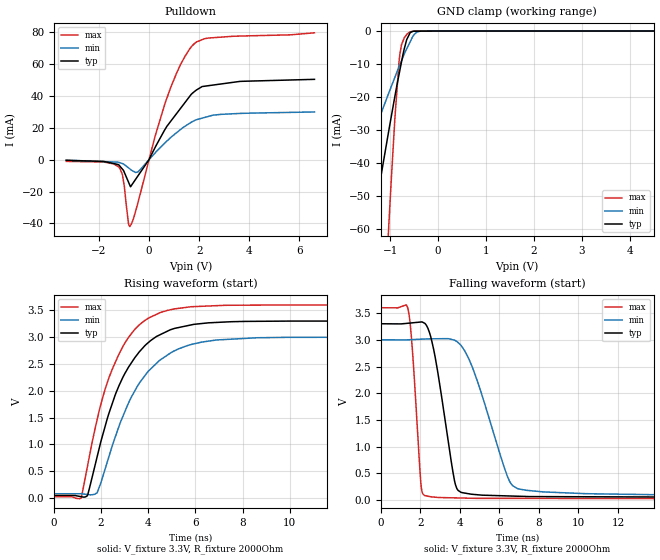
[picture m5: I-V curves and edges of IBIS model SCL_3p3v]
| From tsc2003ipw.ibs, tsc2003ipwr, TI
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|   SCL_3p3v
[Model]   SCL_3p3v
Model_type   I/O_open_drain
Polarity   Non-Inverting
Enable   Active-High
Vinl = 0.99
Vinh = 2.31
Vmeas = 1.65
Vref = 1.65
Cref = 1pF
Rref = 50
|   typ   min   max
C_comp   0.523pF   0.451pF   0.561pF
[Voltage Range]   3.3   3   3.6
[Temperature Range]   27   85   -40
[Pullup Reference]   3.3   3   3.6
[Pulldown Reference]   0   0   0
[Power Clamp Reference]   3.3   3   3.6
[GND Clamp Reference]   0   0   0
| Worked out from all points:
|   slope of the pulldown table from 0 to 0.495 V, typ, clamps not added: 33.1 ohm
|   GND clamp passes 1 mA (typ) near -0.60 V on its own axis
|   falling waveform, V_fixture 3.3V, R_fixture 2000Ohm: 20-80 % time 811ps typ, 1.49ns min, 365ps max; typ from 3.3 V to 0.05 V
|   rising waveform, V_fixture 3.3V, R_fixture 2000Ohm: 20-80 % time 1.69ns typ, 1.87ns min, 1.52ns max; typ from 0.049 V to 3.3 V
[Pulldown]
|   Voltage   I(typ)   I(min)   I(max)
-3.3V     -421.7uA   -283.5uA   -1.075mA
-1.207V   -3.201mA   -1.634mA   -4.56mA
-1.059V   -5.95mA    -2.442mA   -9.342mA
-817.3mV  -14.06mA   -5.123mA   -40.06mA
-764.5mV  -16.01mA   -5.76mA    -42.01mA
-443.3mV  -10.25mA   -7.701mA   -27.15mA
669mV     19.79mA    11.01mA    36.67mA
1.249V    32.01mA    18.82mA    59.44mA
1.771V    42.23mA    24.2mA     72.33mA
2.118V    45.92mA    26.08mA    75.33mA
3.626V    49.15mA    29.04mA    77.61mA
6.6V      50.44mA    29.96mA    79.66mA
[GND Clamp]
|   Voltage   I(typ)   I(min)   I(max)
-3.3V     -229.6mA   -108.6mA   -718.4mA
-2.204V   -132.3mA   -64.83mA   -397.2mA
-2.013V   -115.5mA   -57.24mA   -341.2mA
-1.405V   -62.2mA    -33.27mA   -164.2mA
-1.059V   -32.59mA   -19.88mA   -66.46mA
-1.023V   -29.59mA   -18.52mA   -56.99mA
-905.6mV  -19.99mA   -14.12mA   -26.88mA
-799.7mV  -11.89mA   -10.25mA   -7.023mA
-656.2mV  -2.573mA   -5.357mA   -1.062mA
-555.1mV  -281.6uA   -2.377mA   -123.4uA
-291.9mV  -35.53uA   -1.967uA   0A
6.6V      0A         0A         0A
[POWER Clamp]
|   Voltage   I(typ)   I(min)   I(max)
-3.3V     0A         0A         0A
0V        0A         0A         0A
6.6V      0A         0A         0A
[Ramp]
R_load = 2000
|   typ   min   max
dV/dt_r   1.95079/1.69655e-009   1.75119/1.85441e-009   2.14396/1.51787e-009
dV/dt_f   1.95006/8.10926e-010   1.74662/1.48898e-009   2.14394/3.64926e-010
[Falling Waveform]
V_fixture = 3.3V
V_fixture_min = 3V
V_fixture_max = 3.6V
R_fixture = 2000Ohm
C_fixture = 0F
|   Time   V(typ)   V(min)   V(max)
0s        3.3V       3V         3.6V
1.371ns   3.309V     2.999V     3.594V
1.59ns    3.317V     3.003V     2.871V
2.028ns   3.333V     3.011V     327mV
2.208ns   3.312V     3.014V     89.28mV
2.721ns   2.738V     3.019V     55.82mV
3.734ns   358.7mV    2.993V     42.31mV
4.046ns   148.7mV    2.901V     39.71mV
6.903ns   73.26mV    218.3mV    32.51mV
21.04ns   49.91mV    88.97mV    26.77mV
[Rising Waveform]
V_fixture = 3.3V
V_fixture_min = 3V
V_fixture_max = 3.6V
R_fixture = 2000Ohm
C_fixture = 0F
|   Time   V(typ)   V(min)   V(max)
0s        48.68mV    81.33mV    26.73mV
1.155ns   26.96mV    80.78mV    1.217mV
1.441ns   69.15mV    66.39mV    626.9mV
1.837ns   771.3mV    100.2mV    1.463V
2.344ns   1.59V      785.1mV    2.252V
2.954ns   2.274V     1.551V     2.846V
3.643ns   2.735V     2.154V     3.235V
4.522ns   3.048V     2.578V     3.459V
6.903ns   3.274V     2.947V     3.586V
21.04ns   3.3V       3V         3.6V
